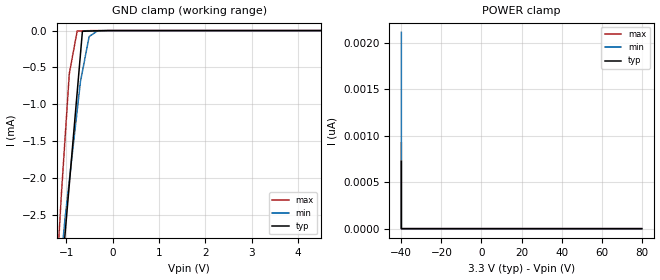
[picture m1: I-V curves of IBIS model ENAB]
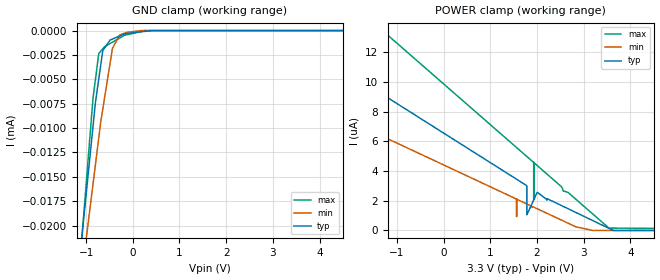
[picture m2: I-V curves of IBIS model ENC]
| Texas Instruments Incorporated
| Mixed Signal Controller
| Marketing part#   Voltage Range   Package-type   Temperature
| TPS43330A-Q1   3V - 3.6V   38-pin HTSSOP   -40 to 150C
[IBIS Ver]   4.0
[File name]   tps43330a.ibs
[File Rev]   1.0
[Date]   08/27/2013
[Source]   Model built from TISPICE simulations at:
   Texas Instruments Incorporated.
   Analog-eLab, HPA
   12500 TI Blvd
   Dallas, TX -75243
   For Support e-mail: elab_scm_ibis@list.ti.com
[Notes]   Rev 1.0: 08/27/2013
   - Model generated from simulations in TISPICED
   - Model not matched to measurements
   - C_comp although listed in numerical order of value are obtained from varying
   PVT conditions. For PVT conditions for each specific value refer the buffer
   description under respective [Model]. IBIS model user is responsible for using
   appropriate C_comp to simulate for Signal Integrity
   Nom PVT:  Nominal process, Typ Temperature, Typ Voltage
   Slow PVT: Weak process, Max Temperature, Min Voltage
   Fast PVT: Strong process, Min Temperatire, Max Voltage
   - POWER clamp non-monotonic warnings for ENC. Behavior based on
   SPICE simulations and accepted.
[Disclaimer] This product is designed as an aid for customers of Texas Instruments.
   No warranties, either expressed or implied, with respect to this third
   party software (if any) or with respect to its fitness for any
   particular purpose is claimed by Texas Instruments or the author. The
   software (if any) is provided solely on an "as is" basis. The entire
   risk as to its quality and performance is with the customer
[Copyright]   (C)Copyright 2013 Texas Instruments Incorporated.
   All rights reserved.
|   TPS43330A DAP
[Component]   TPS43330ADAP
[Manufacturer]  Texas Instruments Incorporated
[Package]   |38-pin DAP
|   typ   min   max
R_pkg   0.0497   0.02154   0.06792
L_pkg   3.0258nH   1.94669nH   4.82882nH
C_pkg   0.4663pF   0.32808pF   0.72166pF
[PIN]   signal_name   model_name   R_pin   L_pin   C_pin
1   VBAT   TERM   0.05608   4.68657n   0.70892p
2   DS   TERM   0.05720   4.06428n   0.63806p
3   GC1   TERM   0.05596   3.45504n   0.49665p
4   GC2   TERM   0.05769   3.01666n   0.40753p
5   CBA   TERM   0.06204   3.03735n   0.41193p
6   GA1   TERM   0.05405   2.72317n   0.41529p
7   PHA   TERM   0.04879   2.50439n   0.40424p
8   GA2   TERM   0.04514   2.34684n   0.35568p
9   PGNDA   GND   0.02185   1.94669n   0.36575p
10   SA1   TERM   0.04046   2.14168n   0.34110p
11   SA2   TERM   0.03992   2.14816n   0.32847p
12   FBA   TERM   0.04161   2.21845n   0.35520p
13   COMPA   TERM   0.04597   2.39975n   0.40972p
14   SSA   TERM   0.05325   2.69229n   0.42553p
15   PGA   TERM   0.06397   3.07269n   0.41524p
16   ENA   ENAB   0.06095   3.14942n   0.41628p
17   ENB   ENAB   0.05315   3.36210n   0.50066p
18   COMPC   TERM   0.05205   3.88801n   0.63329p
19   ENC   ENC   0.05421   4.63512n   0.70347p
20   SYNC   TERM   0.05342   4.60339n   0.70030p
21   DLYAB   TERM   0.05289   3.92201n   0.63474p
22   RT   TERM   0.05420   3.40616n   0.50225p
23   AGND   GND   0.02154   2.76496n   0.46921p
24   PGB   TERM   0.06399   3.08606n   0.41205p
25   SSB   TERM   0.05324   2.66801n   0.40503p
26   COMPB   TERM   0.04598   2.40812n   0.40780p
27   FBB   TERM   0.04161   2.22221n   0.35486p
28   SB2   TERM   0.03993   2.15238n   0.32808p
29   SB1   TERM   0.04046   2.14464n   0.34105p
30   PGNDB   GND   0.02185   1.94882n   0.36578p
31   GB2   TERM   0.04516   2.34085n   0.35954p
32   PHB   TERM   0.04879   2.50000n   0.40946p
33   GB1   TERM   0.05405   2.71774n   0.41589p
34   CBB   TERM   0.06196   3.07640n   0.42118p
35   VREG   TERM   0.03335   2.52829n   0.52499p
36   DIV   TERM   0.06792   3.88970n   0.54342p
37   EXTSUP   TERM   0.06321   4.28177n   0.66801p
38   VIN   POWER   0.05994   4.82882n   0.72166p
|   TERM_3p3v Model
[Model] TERM
Model_type Terminator
C_comp   1fF   1fF   1fF
| variable   typ   min   max
[Voltage Range]   3.3V   3.0V   3.6V
[POWER Clamp Reference]  3.3V   3.0V   3.6V
[GND Clamp Reference]   0.0V   0.0V   0.0V
|Operating Temperature
[Temperature Range]   27   85   -40
| Models and submodels in the file (3): ENAB (Input), ENC (Input), TERM (Terminator)
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|   ENA and ENB Input buffer
[Model]   ENAB
Model_type   Input
|Signals   ENA, ENB
Vinh = 1.7
Vinl = 0.7
|   typ   min   max
|   (typ)   (fast)   (slow)
C_comp   0.891pF   0.824pF   0.924pF
|   typ   min   max
[Temperature Range]   27   -40   150
[Voltage range]   3.3V   3.0V   3.6V
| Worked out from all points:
|   GND clamp passes 1 mA (typ) near -0.78 V on its own axis
| Please note that the voltage is internally regulated, not set by external supply
[GND Clamp]
|   Voltage   I(typ)   I(min)   I(max)
-40V      -499.9mA   -360.5mA   -648.4mA
-1.339V   -5.073mA   -4.686mA   -4.777mA
-1.103V   -3.334mA   -3.077mA   -2.213mA
-1.026V   -2.77mA    -2.555mA   -1.477mA
-932.5mV  -2.085mA   -2.034mA   -582.8uA
-762.5mV  -837uA     -1.083mA   -5.154uA
-693.2mV  -328uA     -695.9uA   -4.167uA
-649.8mV  -8.715uA   -553.5uA   -3.548uA
-505.6mV  -6.468uA   -81.27uA   -1.495uA
-318mV    -3.542uA   -1.34uA    0A
80V       0A         0A         0A
[POWER Clamp]
|   Voltage   I(typ)   I(min)   I(max)
-40V      726.1pA    2.115nA    928.6pA
-40V      0A         0A         0A
-40V      0A         0A         0A
80V       0A         0A         0A
|   ENC buffer
[Model]   ENC
Model_type   Input
|Signals   ENC
Vinh = 1.7
Vinl = 0.7
|   typ   min   max
|   (typ)   (fast)   (slow)
C_comp   0.891pF   0.824pF   0.924pF
|   typ   min   max
[Temperature Range]   27   -40   150
[Voltage range]   3.3V   3.0V   3.6V
| Please note that the voltage is internally regulated, not set by external supply
[GND Clamp]
|   Voltage   I(typ)   I(min)   I(max)
-9V       -427uA     -354.1uA   -547.2uA
-1.217V   -27.15uA   -29.84uA   -28.85uA
-853mV    -9.858uA   -15.77uA   -6.969uA
-801.3mV  -7.403uA   -13.77uA   -5.048uA
-728.7mV  -4.948uA   -10.96uA   -2.35uA
-688.8mV  -3.6uA     -9.423uA   -2.127uA
-643mV    -2.05uA    -8.047uA   -1.87uA
-435.3mV  -865.1nA   -1.812uA   -1.189uA
-278.8mV  -552.3nA   -448.8nA   -760.5nA
-122.3mV  -304.2nA   -177.5nA   -422.8nA
258.4mV   -82.48nA   0A         0A
18V       0A         0A         0A
[POWER Clamp]
|   Voltage   I(typ)   I(min)   I(max)
-9V       58.43uA    20.96uA    98.48uA
-1.757V   10.05uA    6.998uA    14.68uA
1.775V    3.026uA    1.793uA    4.998uA
1.783V    2.995uA    1.781uA    4.977uA
1.783V    2.877uA    1.781uA    4.977uA
1.783V    1.064uA    1.781uA    4.977uA
1.928V    2.053uA    1.574uA    4.577uA
1.929V    2.061uA    1.572uA    4.504uA
1.929V    2.061uA    1.572uA    2.102uA
1.929V    2.064uA    1.571uA    4.598uA
3.196V    662.2nA    0A         1.103uA
18V       0A         0A         0A
